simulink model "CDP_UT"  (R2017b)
settings: Solver=FixedStepDiscrete  StartTime=0.0  StopTime=10.0  FixedStep=0.01  RelTol=1e-3  EnableMultiTasking=on
undefined symbols (not defined in the file): ASWTYPE_FALSE, ASWTYPE_TRUE, CaCDP_CellTempNTCVoltTable_mV, CaCDP_CellTempTable_C, CaCDP_CMUPCBTempNTCVoltTable_mV, CaCDP_CMUPCBTempTable_C, CbCDP_DiffBusbarTempStateCheck_flg, CbCDP_DiffCellTempStateCheck_flg, CbCDP_DiffCellVoltStateCheck_flg, CbCDP_IgnorUpdateVld_flg, CbCDP_MaxBusbarTempStateCheck_flg, CbCDP_MaxCellTempStateCheck_flg, CbCDP_MaxCellVoltStateCheck_flg, CbCDP_MinBusbarTempStateCheck_flg, CbCDP_MinCellTempStateCheck_flg, CbCDP_MinCellVoltStateCheck_flg, CcCDP_AFETempConfig_numb, CcCDP_AFETempFltThd_C, CcCDP_AFETempFltThdHys_C, CcCDP_BusbarTempRngFltHiThrd_C, CcCDP_BusbarTempRngFltLowThrd_C, CcCDP_CellDiffFltLevel1_mV, CcCDP_CellDiffFltLevel2_mV, CcCDP_CellDiffFltLevel3_mV, CcCDP_CellTempLowerLimit_C, CcCDP_CellTempRngFltHiThrd_C, CcCDP_CellTempRngFltLowThrd_C, CcCDP_CellTempUpperLimit_C, CcCDP_CellVoltConfig_numb, CcCDP_CellVoltLowerLimit_mV, CcCDP_CellVoltRngHiThrd_mV, CcCDP_CellVoltRngLowThrd_mV, CcCDP_CellVoltUpdateThrd_numb, CcCDP_CellVoltUpperLimit_mV, CcCDP_ChrgMaxCellTempFltLv1Thrd_C, CcCDP_ChrgMaxCellTempFltLv2Thrd_C, CcCDP_ChrgMaxCellTempFltLv3Thrd_C, CcCDP_ChrgMaxCellTempReturnDiff_C, CcCDP_ChrgMinCellTempFltLv1Thrd_C, CcCDP_ChrgMinCellTempFltLv2Thrd_C, CcCDP_ChrgMinCellTempFltLv3Thrd_C, CcCDP_ChrgMinCellTempReturnDiff_C, CcCDP_CMUPCBTempConfig_numb, CcCDP_CMUPCBTempFltThd_C, CcCDP_CMUPCBTempFltThdHys_C, CcCDP_DiffBusbarTempFltLevel1Thrd_C, CcCDP_DiffBusbarTempFltLevel2Thrd_C, CcCDP_DiffBusbarTempReturnDifference_C, CcCDP_DiffCellTempFltLevel1Thrd_C, CcCDP_DiffCellTempFltLevel2Thrd_C, CcCDP_DiffCellTempReturnDifference_C, CcCDP_DiffCellVoltReturnDifference_mV, CcCDP_DiffVoltCheckMaxCellTempCondition_C, CcCDP_DiffVoltCheckMaxCellVoltCondition_mV, CcCDP_DiffVoltCheckMinCellTempCondition_C, CcCDP_DiffVoltCheckMinCellVoltCondition_mV, CcCDP_DiffVoltCheckPackCurrCondition_A, CcCDP_MaxAFETempIniVal_C, CcCDP_MaxBusbarTempFltLevel1Thrd_C, CcCDP_MaxBusbarTempFltLevel2Thrd_C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
libraries: AIWAYS_Powertrain_BMS_lib x148, simulink x8
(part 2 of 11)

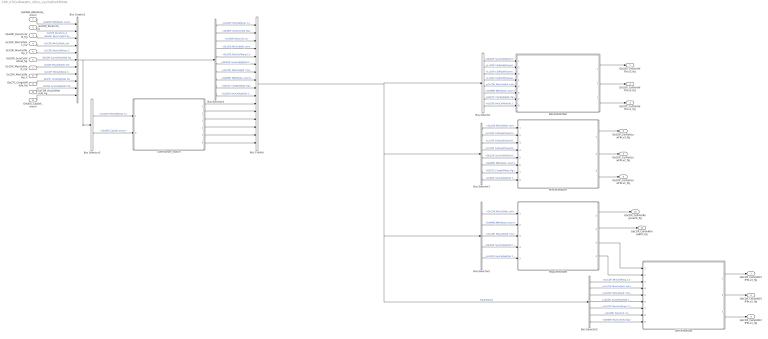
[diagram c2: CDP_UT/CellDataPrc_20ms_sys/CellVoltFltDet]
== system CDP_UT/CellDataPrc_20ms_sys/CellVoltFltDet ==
  GeMSM_BMUState_enum : Inport
  GcHDP_PackCrnt_A : Inport  Port=2
  GbHDP_PackCrntVld_flg : Inport  Port=3
  GcCDP_MinCellVolt_mV : Inport  Port=4
  GcCDP_MaxCellTemp_C : Inport  Port=5
  GbCDP_SumCellVoltVld_flg : Inport  Port=6
  GcCDP_MaxCellVolt_mV : Inport  Port=7
  GcCDP_MinCellTemp_C : Inport  Port=8
  GbCTC_ChrgHVMode_flg : Inport  Port=9
  LbCDP_AnyCellVoltVld_flg : Inport  Port=10
  GeUDS_CapSel_enum : Inport  Port=11
  Bus Creator : BusCreator  Inputs=16
  Bus Creator1 : BusCreator  Inputs=11
  Bus Selector : BusSelector  OutputSignals=GbCDP_SumCellVoltVld_flg,LcCDP_CellHighFltLevel1_mV,LcCDP_CellHighFltLevel2_mV,LcCDP_CellHighFltLevel3_mV,GcCDP_MaxCellVolt_mV,GeMSM_BMUState_enum,GbCTC_ChrgHVMode_flg,LbCDP_AnyCellVoltVld_flg
  Bus Selector1 : BusSelector  OutputSignals=GcCDP_MinCellVolt_mV,LcCDP_CellLowFltLevel1_mV,LcCDP_CellLowFltLevel2_mV,LcCDP_CellLowFltLevel3_mV,GbCDP_SumCellVoltVld_flg,GeMSM_BMUState_enum,GbCTC_ChrgHVMode_flg,LbCDP_AnyCellVoltVld_flg
  Bus Selector2 : BusSelector  OutputSignals=GcCDP_MinCellTemp_C,GcCDP_MaxCellVolt_mV,GcCDP_MinCellVolt_mV,LbCDP_AnyCellVoltVld_flg,GcCDP_MaxCellTemp_C,GcHDP_PackCrnt_A,GbHDP_PackCrntVld_flg
  Bus Selector3 : BusSelector  OutputSignals=GcCDP_MinCellTemp_C,GeUDS_CapSel_enum
  Bus Selector4 : BusSelector  OutputSignals=GcCDP_MinCellTemp_C,GbHDP_PackCrntVld_flg,GcHDP_PackCrnt_A,GcCDP_MinCellVolt_mV,GcCDP_MaxCellTemp_C,GbCDP_SumCellVoltVld_flg,GcCDP_MaxCellVolt_mV,GeMSM_BMUState_enum,GbCTC_ChrgHVMode_flg,LbCDP_AnyCellVoltVld_flg
  Bus Selector5 : BusSelector  OutputSignals=GcCDP_MinCellVolt_mV,GeMSM_BMUState_enum,GcCDP_MaxCellVolt_mV,GbCDP_SumCellVoltVld_flg,LbCDP_AnyCellVoltVld_flg
  CellFltLevel_Switch : Subsystem
  DiffCellVoltDet : Subsystem
  MaxCellVoltDet : Subsystem
  MinCellVoltDet : Subsystem
  RngCellVoltDet : Subsystem
  GbCDP_CellVoltHiFltLv3_flg : Outport
  GbCDP_CellVoltHiFltLv2_flg : Outport  Port=2
  GbCDP_CellVoltHiFltLv1_flg : Outport  Port=3
  GbCDP_CellVoltLowFltLv3_flg : Outport  Port=4
  GbCDP_CellVoltLowFltLv2_flg : Outport  Port=5
  GbCDP_CellVoltLowFltLv1_flg : Outport  Port=6
  GbCDP_CellVoltDiffFltLv3_flg : Outport  Port=7
  GbCDP_CellVoltDiffFltLv2_flg : Outport  Port=8
  GbCDP_CellVoltDiffFltLv1_flg : Outport  Port=9
  GbCDP_CellVoltRngLowFlt_flg : Outport  Port=10
  GbCDP_CellVoltRngHiFlt_flg : Outport  Port=11
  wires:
  Bus Selector4/7 -> Bus Creator/7  "<GcCDP_MaxCellVolt_mV>"
  CellFltLevel_Switch/4(LcCDP_CellLowFltLevel1_mV) -> Bus Creator/14
  CellFltLevel_Switch/2(LcCDP_CellHighFltLevel2_mV) -> Bus Creator/12
  Bus Creator1/1 -> Bus Selector3/1, Bus Selector4/1
  Bus Selector4/3 -> Bus Creator/3  "<GcHDP_PackCrnt_A>"
  Bus Selector4/2 -> Bus Creator/2  "<GbHDP_PackCrntVld_flg>"
  CellFltLevel_Switch/6(LcCDP_CellLowFltLevel3_mV) -> Bus Creator/16
  Bus Selector4/5 -> Bus Creator/5  "<GcCDP_MaxCellTemp_C>"
  CellFltLevel_Switch/1(LcCDP_CellHighFltLevel1_mV) -> Bus Creator/11
  Bus Selector4/8 -> Bus Creator/8  "<GeMSM_BMUState_enum>"
  CellFltLevel_Switch/3(LcCDP_CellHighFltLevel3_mV) -> Bus Creator/13
  Bus Selector4/4 -> Bus Creator/4  "<GcCDP_MinCellVolt_mV>"
  Bus Creator/1 -> Bus Selector2/1, Bus Selector5/1, Bus Selector1/1, Bus Selector/1  "InputSignals"
  Bus Selector3/1 -> CellFltLevel_Switch/1(GcCDP_MinCellTemp_C)  "<GcCDP_MinCellTemp_C>"
  Bus Selector4/1 -> Bus Creator/1  "<GcCDP_MinCellTemp_C>"
  CellFltLevel_Switch/5(LcCDP_CellLowFltLevel2_mV) -> Bus Creator/15
  Bus Selector4/6 -> Bus Creator/6  "<GbCDP_SumCellVoltVld_flg>"
  GeMSM_BMUState_enum/1 -> Bus Creator1/1  "GeMSM_BMUState_enum"
  GcHDP_PackCrnt_A/1 -> Bus Creator1/2  "GcHDP_PackCrnt_A"
  GbHDP_PackCrntVld_flg/1 -> Bus Creator1/3  "GbHDP_PackCrntVld_flg"
  GcCDP_MinCellVolt_mV/1 -> Bus Creator1/4  "GcCDP_MinCellVolt_mV"
  GcCDP_MaxCellTemp_C/1 -> Bus Creator1/5  "GcCDP_MaxCellTemp_C"
  GbCDP_SumCellVoltVld_flg/1 -> Bus Creator1/6  "GbCDP_SumCellVoltVld_flg"
  GcCDP_MaxCellVolt_mV/1 -> Bus Creator1/7  "GcCDP_MaxCellVolt_mV"
  GcCDP_MinCellTemp_C/1 -> Bus Creator1/8  "GcCDP_MinCellTemp_C"
  GbCTC_ChrgHVMode_flg/1 -> Bus Creator1/9  "GbCTC_ChrgHVMode_flg"
  Bus Selector4/9 -> Bus Creator/9  "<GbCTC_ChrgHVMode_flg>"
  MaxCellVoltDet/1(GbCDP_CellVoltHiFltLv3_flg) -> GbCDP_CellVoltHiFltLv3_flg/1
  MaxCellVoltDet/2(GbCDP_CellVoltHiFltLv2_flg) -> GbCDP_CellVoltHiFltLv2_flg/1
  MaxCellVoltDet/3(GbCDP_CellVoltHiFltLv1_flg) -> GbCDP_CellVoltHiFltLv1_flg/1
  MinCellVoltDet/1(GbCDP_CellVoltLowFltLv3_flg) -> GbCDP_CellVoltLowFltLv3_flg/1
  MinCellVoltDet/2(GbCDP_CellVoltLowFltLv2_flg) -> GbCDP_CellVoltLowFltLv2_flg/1
  MinCellVoltDet/3(GbCDP_CellVoltLowFltLv1_flg) -> GbCDP_CellVoltLowFltLv1_flg/1
  DiffCellVoltDet/1(GbCDP_CellVoltDiffFltLv3_flg) -> GbCDP_CellVoltDiffFltLv3_flg/1
  DiffCellVoltDet/2(GbCDP_CellVoltDiffFltLv2_flg) -> GbCDP_CellVoltDiffFltLv2_flg/1
  DiffCellVoltDet/3(GbCDP_CellVoltDiffFltLv1_flg) -> GbCDP_CellVoltDiffFltLv1_flg/1
  Bus Selector5/1 -> RngCellVoltDet/1(GcCDP_MinCellVolt_mV)  "<GcCDP_MinCellVolt_mV>"
  Bus Selector5/2 -> RngCellVoltDet/2(GeMSM_BMUState_enum)  "<GeMSM_BMUState_enum>"
  Bus Selector5/3 -> RngCellVoltDet/3(GcCDP_MaxCellVolt_mV)  "<GcCDP_MaxCellVolt_mV>"
  Bus Selector5/4 -> RngCellVoltDet/4(GbCDP_SumCellVoltVld_flg)  "<GbCDP_SumCellVoltVld_flg>"
  RngCellVoltDet/1(GbCDP_CellVoltRngLowFlt_flg) -> GbCDP_CellVoltRngLowFlt_flg/1
  RngCellVoltDet/2(GbCDP_CellVoltRngHiFlt_flg) -> GbCDP_CellVoltRngHiFlt_flg/1
  LbCDP_AnyCellVoltVld_flg/1 -> Bus Creator1/10  "LbCDP_AnyCellVoltVld_flg"
  Bus Selector4/10 -> Bus Creator/10  "<LbCDP_AnyCellVoltVld_flg>"
  Bus Selector5/5 -> RngCellVoltDet/5(LbCDP_AnyCellVoltVld_flg)  "<LbCDP_AnyCellVoltVld_flg>"
  Bus Selector/1 -> MaxCellVoltDet/1(GbCDP_SumCellVoltVld_flg)  "<GbCDP_SumCellVoltVld_flg>"
  Bus Selector/2 -> MaxCellVoltDet/2(LcCDP_CellHighFltLevel1_mV)  "<LcCDP_CellHighFltLevel1_mV>"
  Bus Selector/3 -> MaxCellVoltDet/3(LcCDP_CellHighFltLevel2_mV)  "<LcCDP_CellHighFltLevel2_mV>"
  Bus Selector/4 -> MaxCellVoltDet/4(LcCDP_CellHighFltLevel3_mV)  "<LcCDP_CellHighFltLevel3_mV>"
  Bus Selector/5 -> MaxCellVoltDet/5(GcCDP_MaxCellVolt_mV)  "<GcCDP_MaxCellVolt_mV>"
  Bus Selector/6 -> MaxCellVoltDet/6(GeMSM_BMUState_enum)  "<GeMSM_BMUState_enum>"
  Bus Selector/7 -> MaxCellVoltDet/7(GbCTC_ChrgHVMode_flg)  "<GbCTC_ChrgHVMode_flg>"
  Bus Selector/8 -> MaxCellVoltDet/8(LbCDP_AnyCellVoltVld_flg)  "<LbCDP_AnyCellVoltVld_flg>"
  Bus Selector1/1 -> MinCellVoltDet/1(GcCDP_MinCellVolt_mV)  "<GcCDP_MinCellVolt_mV>"
  Bus Selector1/2 -> MinCellVoltDet/2(LcCDP_CellLowFltLevel1_mV)  "<LcCDP_CellLowFltLevel1_mV>"
  Bus Selector1/3 -> MinCellVoltDet/3(LcCDP_CellLowFltLevel2_mV)  "<LcCDP_CellLowFltLevel2_mV>"
  Bus Selector1/4 -> MinCellVoltDet/4(LcCDP_CellLowFltLevel3_mV)  "<LcCDP_CellLowFltLevel3_mV>"
  Bus Selector1/5 -> MinCellVoltDet/5(GbCDP_SumCellVoltVld_flg)  "<GbCDP_SumCellVoltVld_flg>"
  Bus Selector1/6 -> MinCellVoltDet/6(GeMSM_BMUState_enum)  "<GeMSM_BMUState_enum>"
  Bus Selector1/7 -> MinCellVoltDet/7(GbCTC_ChrgHVMode_flg)  "<GbCTC_ChrgHVMode_flg>"
  Bus Selector1/8 -> MinCellVoltDet/8(LbCDP_AnyCellVoltVld_flg)  "<LbCDP_AnyCellVoltVld_flg>"
  Bus Selector2/1 -> DiffCellVoltDet/3(GcCDP_MinCellTemp_C)  "<GcCDP_MinCellTemp_C>"
  Bus Selector2/2 -> DiffCellVoltDet/4(GcCDP_MaxCellVolt_mV)  "<GcCDP_MaxCellVolt_mV>"
  Bus Selector2/3 -> DiffCellVoltDet/5(GcCDP_MinCellVolt_mV)  "<GcCDP_MinCellVolt_mV>"
  Bus Selector2/4 -> DiffCellVoltDet/6(LbCDP_AnyCellVoltVld_flg)  "<LbCDP_AnyCellVoltVld_flg>"
  Bus Selector2/5 -> DiffCellVoltDet/7(GcCDP_MaxCellTemp_C)  "<GcCDP_MaxCellTemp_C>"
  Bus Selector2/6 -> DiffCellVoltDet/8(GcHDP_PackCrnt_A)  "<GcHDP_PackCrnt_A>"
  Bus Selector2/7 -> DiffCellVoltDet/9(GbHDP_PackCrntVld_flg)  "<GbHDP_PackCrntVld_flg>"
  RngCellVoltDet/3(LbCDP_CellVoltRngLowFlt_flg) -> DiffCellVoltDet/1(LbCDP_CellVoltRngLowFlt_flg)
  RngCellVoltDet/4(LbCDP_CellVoltRngHiFlt_flg) -> DiffCellVoltDet/2(LbCDP_CellVoltRngHiFlt_flg)
  GeUDS_CapSel_enum/1 -> Bus Creator1/11
  Bus Selector3/2 -> CellFltLevel_Switch/2(GeUDS_CapSel_enum)  "<GeUDS_CapSel_enum>"

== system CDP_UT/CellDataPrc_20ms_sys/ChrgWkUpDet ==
  GeCTC_CtrCtlConnMode_enum : Inport
  Comparison1 : RelationalOperator  Operator===  OutDataTypeStr=boolean
  Comparison2 : RelationalOperator  Operator===  OutDataTypeStr=boolean
  Constant2 : Constant  Value=Enum_CTCCtrCtlConnMode.Enum_CTCCtrCtlConnMode_ACChrg
  Constant3 : Constant  Value=Enum_CTCCtrCtlConnMode.Enum_CTCCtrCtlConnMode_DCChrg
  Data Type Conversion : DataTypeConversion
  Logical1 : Logic  Operator=OR  OutDataTypeStr=boolean
  LbCDP_ChrgWkUp_flg : Outport
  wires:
  GeCTC_CtrCtlConnMode_enum/1 -> Data Type Conversion/1
  Constant2/1 -> Comparison1/2
  Logical1/1 -> LbCDP_ChrgWkUp_flg/1  "LbCDP_ChrgWkUp_flg"
  Constant3/1 -> Comparison2/1
  Comparison2/1 -> Logical1/1
  Comparison1/1 -> Logical1/2
  Data Type Conversion/1 -> Comparison1/1, Comparison2/2

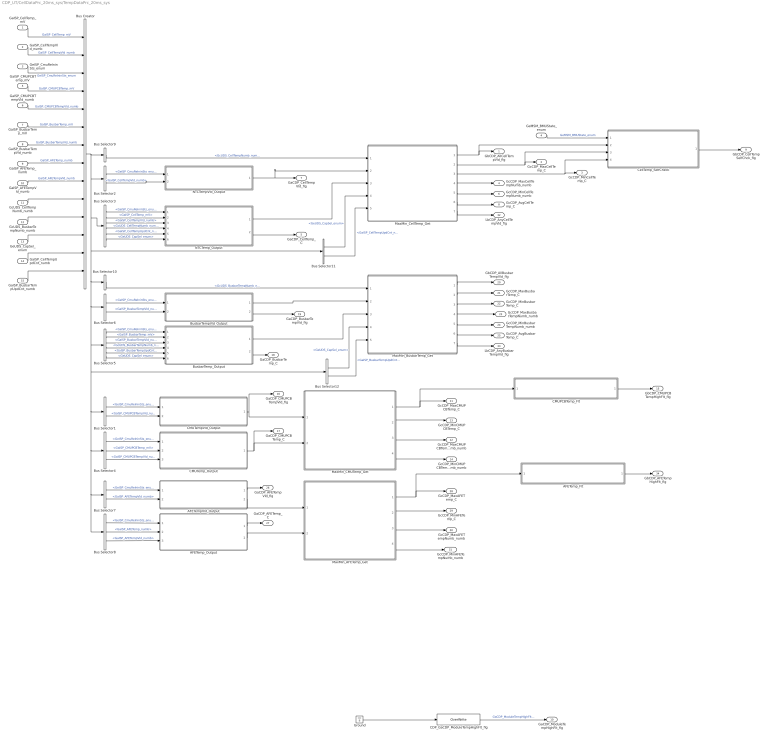
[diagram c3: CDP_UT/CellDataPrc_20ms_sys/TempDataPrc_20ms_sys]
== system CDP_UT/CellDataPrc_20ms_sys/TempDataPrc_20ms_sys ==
  GaISP_CellTemp_mV : Inport
  GaISP_CellTempVld_numb : Inport  Port=2
  GeISP_CmuReIninSts_enum : Inport  Port=3
  GeMSM_BMUState_enum : Inport  Port=4
  GaISP_CMUPCBTemp_mV : Inport  Port=5
  GaISP_CMUPCBTempVld_numb : Inport  Port=6
  GaISP_BusbarTemp_mV : Inport  Port=7
  GaISP_BusbarTempVld_numb : Inport  Port=8
  GaISP_AFETemp_numb : Inport  Port=9
  GaISP_AFETempVld_numb : Inport  Port=10
  GcUDS_CellTempNumb_numb : Inport  Port=11
  GcUDS_BusbarTempNumb_numb : Inport  Port=12
  GeUDS_CapSel_enum : Inport  Port=13
  GaISP_CellTempUpdCnt_numb : Inport  Port=14
  GaISP_BusbarTempUpdCnt_numb : Inport  Port=15
  AFETempVld_Output : Subsystem
  AFETemp_Flt : Subsystem
  AFETemp_Output : Subsystem
  Bus Creator : BusCreator  Inputs=14
  Bus Selector1 : BusSelector  OutputSignals=GeISP_CmuReIninSts_enum,GaISP_CMUPCBTempVld_numb
  Bus Selector10 : BusSelector  OutputSignals=GcUDS_BusbarTempNumb_numb
  Bus Selector11 : BusSelector  OutputSignals=GeUDS_CapSel_enum,GaISP_CellTempUpdCnt_numb
  Bus Selector12 : BusSelector  OutputSignals=GeUDS_CapSel_enum,GaISP_BusbarTempUpdCnt_numb
  Bus Selector2 : BusSelector  OutputSignals=GeISP_CmuReIninSts_enum,GaISP_CellTempVld_numb
  Bus Selector3 : BusSelector  OutputSignals=GeISP_CmuReIninSts_enum,GaISP_CellTemp_mV,GaISP_CellTempVld_numb,GcUDS_CellTempNumb_numb,GaISP_CellTempUpdCnt_numb,GeUDS_CapSel_enum
  Bus Selector4 : BusSelector  OutputSignals=GeISP_CmuReIninSts_enum,GaISP_CMUPCBTemp_mV,GaISP_CMUPCBTempVld_numb
  Bus Selector5 : BusSelector  OutputSignals=GeISP_CmuReIninSts_enum,GaISP_BusbarTemp_mV,GaISP_BusbarTempVld_numb,GcUDS_BusbarTempNumb_numb,GaISP_BusbarTempUpdCnt_numb,GeUDS_CapSel_enum
  Bus Selector6 : BusSelector  OutputSignals=GeISP_CmuReIninSts_enum,GaISP_BusbarTempVld_numb
  Bus Selector7 : BusSelector  OutputSignals=GeISP_CmuReIninSts_enum,GaISP_AFETempVld_numb
  Bus Selector8 : BusSelector  OutputSignals=GeISP_CmuReIninSts_enum,GaISP_AFETemp_numb,GaISP_AFETempVld_numb
  Bus Selector9 : BusSelector  OutputSignals=GcUDS_CellTempNumb_numb
  BusbarTempVld_Output : Subsystem
  BusbarTemp_Output : Subsystem
  CDP_GaCDP_ModuleTempHighFlt_flg : AIWAYS_Powertrain_BMS_lib/Signals/OverWrite  OverWrite_Value=CaCDP_ModuleTempHighFltOvr_flg  OverWrite_flag=CbCDP_ModuleTempHighFltOvrSwt_flg
  CMUPCBTemp_Flt : Subsystem
  CMUTempVld_Output : Subsystem
  CMUTemp_Output : Subsystem
  CellTemp_SelfCheck : Subsystem
  Ground : Ground
  MaxMin_AFETemp_Get : Subsystem
  MaxMin_BusbarTemp_Get : Subsystem
  MaxMin_CMUTemp_Get : Subsystem
  MaxMin_CellTemp_Get : Subsystem
  NTCTempVld_Output : Subsystem
  NTCTemp_Output : Subsystem
  GbCDP_AllCellTempVld_flg : Outport
  GcCDP_MaxCellTemp_C : Outport  Port=2
  GcCDP_MinCellTemp_C : Outport  Port=3
  GcCDP_MaxCellTempNumb_numb : Outport  Port=4
  GaCDP_CellTemp_C : Outport  Port=5
  GcCDP_MinCellTempNumb_numb : Outport  Port=6
  GaCDP_CellTempVld_flg : Outport  Port=7
  GcCDP_AvgCellTemp_C : Outport  Port=8
  GbCDP_CellTempSelfChck_flg : Outport  Port=9
  GaCDP_ModuleTempHighFlt_flg : Outport  Port=10
  GcCDP_MaxCMUPCBTemp_C : Outport  Port=11
  GcCDP_MaxCMUPCBTempNumb_numb : Outport  Port=12
  GcCDP_MinCMUPCBTemp_C : Outport  Port=13
  GcCDP_MinCMUPCBTempNumb_numb : Outport  Port=14
  GbCDP_CMUPCBTempHighFlt_flg : Outport  Port=15
  GaCDP_CMUPCBTempVld_flg : Outport  Port=16
  GaCDP_CMUPCBTemp_C : Outport  Port=17
  GaCDP_BusbarTemp_C : Outport  Port=18
  GaCDP_BusbarTempVld_flg : Outport  Port=19
  GbCDP_AllBusbarTempVld_flg : Outport  Port=20
  GcCDP_MaxBusbarTemp_C : Outport  Port=21
  GcCDP_MinBusbarTemp_C : Outport  Port=22
  GcCDP_MaxBusbarTempNumb_numb : Outport  Port=23
  GcCDP_MinBusbarTempNumb_numb : Outport  Port=24
  GcCDP_AvgBusbarTemp_C : Outport  Port=25
  GaCDP_AFETempVld_flg : Outport  Port=26
  GaCDP_AFETemp_C : Outport  Port=27
  GcCDP_MaxAFETemp_C : Outport  Port=28
  GcCDP_MinAFETemp_C : Outport  Port=29
  GcCDP_MaxAFETempNumb_numb : Outport  Port=30
  GcCDP_MinAFETempNumb_numb : Outport  Port=31
  LbCDP_AnyCellTempVld_flg : Outport  Port=32
  LbCDP_AnyBusbarTempVld_flg : Outport  Port=33
  GbCDP_AFETempHighFlt_flg : Outport  Port=34
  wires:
  GaISP_CellTemp_mV/1 -> Bus Creator/1  "GaISP_CellTemp_mV"
  GeISP_CmuReIninSts_enum/1 -> Bus Creator/3  "GeISP_CmuReIninSts_enum"
  MaxMin_CellTemp_Get/5(GcCDP_MinCellTempNumb_numb) -> GcCDP_MinCellTempNumb_numb/1
  MaxMin_CellTemp_Get/6(GcCDP_AvgCellTemp_C) -> GcCDP_AvgCellTemp_C/1
  GaISP_CellTempVld_numb/1 -> Bus Creator/2  "GaISP_CellTempVld_numb"
  MaxMin_CellTemp_Get/3(GcCDP_MinCellTemp_C) -> CellTemp_SelfCheck/4(GcCDP_MinCellTemp_C), GcCDP_MinCellTemp_C/1
  MaxMin_CellTemp_Get/2(GcCDP_MaxCellTemp_C) -> CellTemp_SelfCheck/3(GcCDP_MaxCellTemp_C), GcCDP_MaxCellTemp_C/1
  MaxMin_CellTemp_Get/1(GbCDP_AllCellTempVld_flg) -> CellTemp_SelfCheck/2(GbCDP_AllCellTempVld_flg), GbCDP_AllCellTempVld_flg/1
  MaxMin_CellTemp_Get/4(GcCDP_MaxCellTempNumb_numb) -> GcCDP_MaxCellTempNumb_numb/1
  NTCTempVld_Output/1(GaCDP_CellTempVld_flg) -> MaxMin_CellTemp_Get/2(GaCDP_CellTempVld_flg), GaCDP_CellTempVld_flg/1
  Bus Selector2/1 -> NTCTempVld_Output/1(GeISP_CmuReIninSts_enum)  "<GeISP_CmuReIninSts_enum>"
  Bus Selector2/2 -> NTCTempVld_Output/2(GaISP_CellTempVld_numb)  "<GaISP_CellTempVld_numb>"
  Bus Selector3/2 -> NTCTemp_Output/2(GaISP_CellTemp_mV)  "<GaISP_CellTemp_mV>"
  Bus Selector3/1 -> NTCTemp_Output/1(GeISP_CmuReIninSts_enum)  "<GeISP_CmuReIninSts_enum>"
  Bus Selector3/3 -> NTCTemp_Output/3(GaISP_CellTempVld_numb)  "<GaISP_CellTempVld_numb>"
  CellTemp_SelfCheck/1(GbCDP_CellTempSelfChck_flg) -> GbCDP_CellTempSelfChck_flg/1
  GeMSM_BMUState_enum/1 -> CellTemp_SelfCheck/1(GeMSM_BMUState_enum)  "GeMSM_BMUState_enum"
  GaISP_CMUPCBTemp_mV/1 -> Bus Creator/4  "GaISP_CMUPCBTemp_mV"
  GaISP_CMUPCBTempVld_numb/1 -> Bus Creator/5  "GaISP_CMUPCBTempVld_numb"
  CDP_GaCDP_ModuleTempHighFlt_flg/1 -> GaCDP_ModuleTempHighFlt_flg/1  "GaCDP_ModuleTempHighFlt_flg"
  Ground/1 -> CDP_GaCDP_ModuleTempHighFlt_flg/1
  CMUTemp_Output/1(GaCDP_CMUPCBTemp_C) -> MaxMin_CMUTemp_Get/2(GaCDP_CMUPCBTemp_C), GaCDP_CMUPCBTemp_C/1
  Bus Selector1/1 -> CMUTempVld_Output/1(GeISP_CmuReIninSts_enum)  "<GeISP_CmuReIninSts_enum>"
  Bus Selector4/1 -> CMUTemp_Output/1(GeISP_CmuReIninSts_enum)  "<GeISP_CmuReIninSts_enum>"
  Bus Selector4/3 -> CMUTemp_Output/3(GaISP_CMUPCBTempVld_numb)  "<GaISP_CMUPCBTempVld_numb>"
  Bus Selector4/2 -> CMUTemp_Output/2(GaISP_CMUPCBTemp_mV)  "<GaISP_CMUPCBTemp_mV>"
  CMUTempVld_Output/1(GaCDP_CMUPCBTempVld_flg) -> MaxMin_CMUTemp_Get/1(GaCDP_CMUPCBTempVld_flg), GaCDP_CMUPCBTempVld_flg/1
  Bus Selector1/2 -> CMUTempVld_Output/2(GaISP_CMUPCBTempVld_numb)  "<GaISP_CMUPCBTempVld_numb>"
  MaxMin_CMUTemp_Get/1(GcCDP_MaxCMUPCBTemp_C) -> CMUPCBTemp_Flt/1(GcCDP_MaxCMUPCBTemp_C), GcCDP_MaxCMUPCBTemp_C/1
  CMUPCBTemp_Flt/1(GbCDP_CMUPCBTempHighFlt_flg) -> GbCDP_CMUPCBTempHighFlt_flg/1
  MaxMin_CMUTemp_Get/2(GcCDP_MinCMUPCBTemp_C) -> GcCDP_MinCMUPCBTemp_C/1
  MaxMin_CMUTemp_Get/3(GcCDP_MaxCMUPCBTempNumb_numb) -> GcCDP_MaxCMUPCBTempNumb_numb/1
  MaxMin_CMUTemp_Get/4(GcCDP_MinCMUPCBTempNumb_numb) -> GcCDP_MinCMUPCBTempNumb_numb/1
  GaISP_BusbarTemp_mV/1 -> Bus Creator/6  "GaISP_BusbarTemp_mV"
  GaISP_BusbarTempVld_numb/1 -> Bus Creator/7  "GaISP_BusbarTempVld_numb"
  Bus Selector6/1 -> BusbarTempVld_Output/1(GeISP_CmuReIninSts_enum)  "<GeISP_CmuReIninSts_enum>"
  Bus Selector6/2 -> BusbarTempVld_Output/2(GaISP_BusbarTempVld_numb)  "<GaISP_BusbarTempVld_numb>"
  Bus Selector5/1 -> BusbarTemp_Output/1(GeISP_CmuReIninSts_enum)  "<GeISP_CmuReIninSts_enum>"
  Bus Selector5/2 -> BusbarTemp_Output/2(GaISP_BusbarTemp_mV)  "<GaISP_BusbarTemp_mV>"
  Bus Selector5/3 -> BusbarTemp_Output/3(GaISP_BusbarTempVld_numb)  "<GaISP_BusbarTempVld_numb>"
  BusbarTemp_Output/1(LaCDP_BusbarTemp_C) -> MaxMin_BusbarTemp_Get/3(LaCDP_BusbarTemp_C)
  BusbarTempVld_Output/2(GaCDP_BusbarTempVld_flg) -> GaCDP_BusbarTempVld_flg/1
  BusbarTemp_Output/2(GaCDP_BusbarTemp_C) -> GaCDP_BusbarTemp_C/1
  BusbarTempVld_Output/1(LaCDP_BusbarTempVld_flg) -> MaxMin_BusbarTemp_Get/2(LaCDP_BusbarTempVld_flg)
  MaxMin_BusbarTemp_Get/1(GbCDP_AllBusbarTempVld_flg) -> GbCDP_AllBusbarTempVld_flg/1
  MaxMin_BusbarTemp_Get/2(GcCDP_MaxBusbarTemp_C) -> GcCDP_MaxBusbarTemp_C/1
  MaxMin_BusbarTemp_Get/3(GcCDP_MinBusbarTemp_C) -> GcCDP_MinBusbarTemp_C/1
  MaxMin_BusbarTemp_Get/4(GcCDP_MaxBusbarTempNumb_numb) -> GcCDP_MaxBusbarTempNumb_numb/1
  MaxMin_BusbarTemp_Get/5(GcCDP_MinBusbarTempNumb_numb) -> GcCDP_MinBusbarTempNumb_numb/1
  MaxMin_BusbarTemp_Get/6(GcCDP_AvgBusbarTemp_C) -> GcCDP_AvgBusbarTemp_C/1
  GaISP_AFETemp_numb/1 -> Bus Creator/8  "GaISP_AFETemp_numb"
  GaISP_AFETempVld_numb/1 -> Bus Creator/9  "GaISP_AFETempVld_numb"
  Bus Selector7/1 -> AFETempVld_Output/1(GeISP_CmuReIninSts_enum)  "<GeISP_CmuReIninSts_enum>"
  Bus Selector7/2 -> AFETempVld_Output/2(GaISP_AFETempVld_numb)  "<GaISP_AFETempVld_numb>"
  Bus Selector8/1 -> AFETemp_Output/1(GeISP_CmuReIninSts_enum)  "<GeISP_CmuReIninSts_enum>"
  Bus Selector8/2 -> AFETemp_Output/2(GaISP_AFETemp_numb)  "<GaISP_AFETemp_numb>"
  Bus Selector8/3 -> AFETemp_Output/3(GaISP_AFETempVld_numb)  "<GaISP_AFETempVld_numb>"
  AFETemp_Output/2(LaCDP_AFETemp_C) -> MaxMin_AFETemp_Get/2(LaCDP_AFETemp_C)
  AFETempVld_Output/2(LaCDP_AFETempVld_flg) -> MaxMin_AFETemp_Get/1(LaCDP_AFETempVld_flg)
  AFETempVld_Output/1(GaCDP_AFETempVld_flg) -> GaCDP_AFETempVld_flg/1
  AFETemp_Output/1(GaCDP_AFETemp_C) -> GaCDP_AFETemp_C/1
  MaxMin_AFETemp_Get/1(GcCDP_MaxAFETemp_C) -> AFETemp_Flt/1(GcCDP_MaxAFETemp_C), GcCDP_MaxAFETemp_C/1
  MaxMin_AFETemp_Get/2(GcCDP_MinAFETemp_C) -> GcCDP_MinAFETemp_C/1
  MaxMin_AFETemp_Get/3(GcCDP_MaxAFETempNumb_numb) -> GcCDP_MaxAFETempNumb_numb/1
  MaxMin_AFETemp_Get/4(GcCDP_MinAFETempNumb_numb) -> GcCDP_MinAFETempNumb_numb/1
  MaxMin_CellTemp_Get/7(LbCDP_AnyCellTempVld_flg) -> LbCDP_AnyCellTempVld_flg/1
  MaxMin_BusbarTemp_Get/7(LbCDP_AnyBusbarTempVld_flg) -> LbCDP_AnyBusbarTempVld_flg/1
  GcUDS_CellTempNumb_numb/1 -> Bus Creator/10
  GcUDS_BusbarTempNumb_numb/1 -> Bus Creator/11
  Bus Creator/1 -> Bus Selector11/1, Bus Selector12/1, Bus Selector8/1, Bus Selector7/1, Bus Selector4/1, Bus Selector1/1, Bus Selector5/1, Bus Selector6/1, Bus Selector10/1, Bus Selector3/1, Bus Selector2/1, Bus Selector9/1
  Bus Selector10/1 -> MaxMin_BusbarTemp_Get/1(GcUDS_BusbarTempNumb_numb)  "<GcUDS_BusbarTempNumb_numb>"
  Bus Selector9/1 -> MaxMin_CellTemp_Get/1(GcUDS_CellTempNumb_numb)  "<GcUDS_CellTempNumb_numb>"
  Bus Selector5/4 -> BusbarTemp_Output/4(GcUDS_BusbarTempNumb_numb)  "<GcUDS_BusbarTempNumb_numb>"
  Bus Selector3/4 -> NTCTemp_Output/4(GcUDS_CellTempNumb_numb)  "<GcUDS_CellTempNumb_numb>"
  AFETemp_Flt/1(GbCDP_AFETempHighFlt_flg) -> GbCDP_AFETempHighFlt_flg/1
  GeUDS_CapSel_enum/1 -> Bus Creator/12
  GaISP_CellTempUpdCnt_numb/1 -> Bus Creator/13
  Bus Selector11/1 -> MaxMin_CellTemp_Get/4(GeUDS_CapSel_enum)  "<GeUDS_CapSel_enum>"
  Bus Selector11/2 -> MaxMin_CellTemp_Get/5(GaISP_CellTempUpdCnt_numb)  "<GaISP_CellTempUpdCnt_numb>"
  NTCTemp_Output/1(LaCDP_CellTemp_C) -> MaxMin_CellTemp_Get/3(LaCDP_CellTemp_C)
  NTCTemp_Output/2(GaCDP_CellTemp_C) -> GaCDP_CellTemp_C/1
  Bus Selector3/5 -> NTCTemp_Output/5(GaISP_CellTempUpdCnt_numb)  "<GaISP_CellTempUpdCnt_numb>"
  Bus Selector3/6 -> NTCTemp_Output/6(GeUDS_CapSel_enum)  "<GeUDS_CapSel_enum>"
  GaISP_BusbarTempUpdCnt_numb/1 -> Bus Creator/14
  Bus Selector5/5 -> BusbarTemp_Output/5(GaISP_BusbarTempUpdCnt_numb)  "<GaISP_BusbarTempUpdCnt_numb>"
  Bus Selector5/6 -> BusbarTemp_Output/6(GeUDS_CapSel_enum)  "<GeUDS_CapSel_enum>"
  Bus Selector12/1 -> MaxMin_BusbarTemp_Get/4(GeUDS_CapSel_enum)  "<GeUDS_CapSel_enum>"
  Bus Selector12/2 -> MaxMin_BusbarTemp_Get/5(GaISP_BusbarTempUpdCnt_numb)  "<GaISP_BusbarTempUpdCnt_numb>"

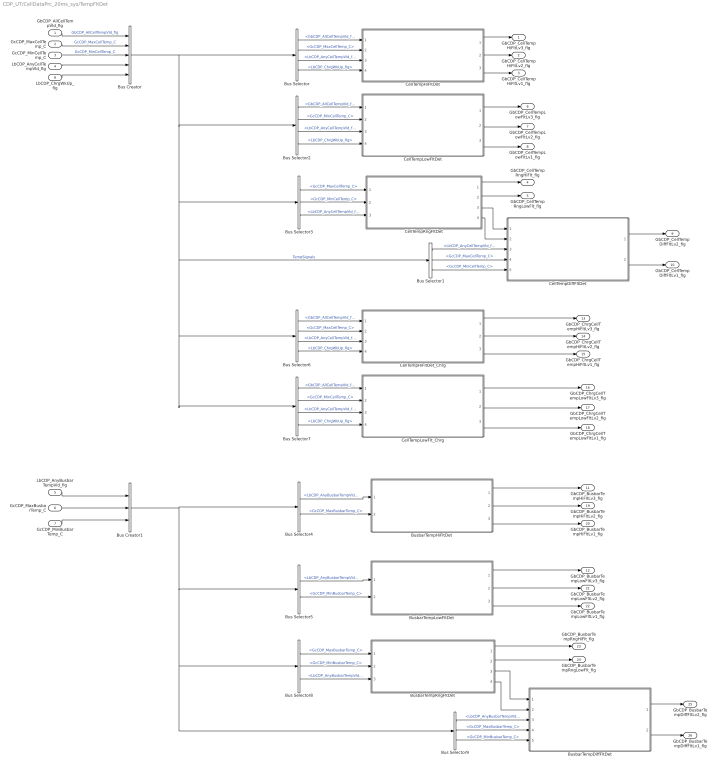
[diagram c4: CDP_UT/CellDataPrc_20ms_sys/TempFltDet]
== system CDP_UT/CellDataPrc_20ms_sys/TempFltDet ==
  GbCDP_AllCellTempVld_flg : Inport
  GcCDP_MaxCellTemp_C : Inport  Port=2
  GcCDP_MinCellTemp_C : Inport  Port=3
  LbCDP_AnyCellTempVld_flg : Inport  Port=4
  LbCDP_AnyBusbarTempVld_flg : Inport  Port=5
  GcCDP_MaxBusbarTemp_C : Inport  Port=6
  GcCDP_MinBusbarTemp_C : Inport  Port=7
  LbCDP_ChrgWkUp_flg : Inport  Port=8
  Bus Creator : BusCreator  Inputs=5
  Bus Creator1 : BusCreator  Inputs=3
  Bus Selector : BusSelector  OutputSignals=GbCDP_AllCellTempVld_flg,GcCDP_MaxCellTemp_C,LbCDP_AnyCellTempVld_flg,LbCDP_ChrgWkUp_flg
  Bus Selector1 : BusSelector  OutputSignals=LbCDP_AnyCellTempVld_flg,GcCDP_MaxCellTemp_C,GcCDP_MinCellTemp_C
  Bus Selector2 : BusSelector  OutputSignals=GbCDP_AllCellTempVld_flg,GcCDP_MinCellTemp_C,LbCDP_AnyCellTempVld_flg,LbCDP_ChrgWkUp_flg
  Bus Selector3 : BusSelector  OutputSignals=GcCDP_MaxCellTemp_C,GcCDP_MinCellTemp_C,LbCDP_AnyCellTempVld_flg
  Bus Selector4 : BusSelector  OutputSignals=LbCDP_AnyBusbarTempVld_flg,GcCDP_MaxBusbarTemp_C
  Bus Selector5 : BusSelector  OutputSignals=LbCDP_AnyBusbarTempVld_flg,GcCDP_MinBusbarTemp_C
  Bus Selector6 : BusSelector  OutputSignals=GbCDP_AllCellTempVld_flg,GcCDP_MaxCellTemp_C,LbCDP_AnyCellTempVld_flg,LbCDP_ChrgWkUp_flg
  Bus Selector7 : BusSelector  OutputSignals=GbCDP_AllCellTempVld_flg,GcCDP_MinCellTemp_C,LbCDP_AnyCellTempVld_flg,LbCDP_ChrgWkUp_flg
  Bus Selector8 : BusSelector  OutputSignals=GcCDP_MaxBusbarTemp_C,GcCDP_MinBusbarTemp_C,LbCDP_AnyBusbarTempVld_flg
  Bus Selector9 : BusSelector  OutputSignals=LbCDP_AnyBusbarTempVld_flg,GcCDP_MaxBusbarTemp_C,GcCDP_MinBusbarTemp_C
  BusbarTempDiffFltDet : Subsystem
  BusbarTempHiFltDet : Subsystem
  BusbarTempLowFltDet : Subsystem
  BusbarTempRngFltDet : Subsystem
  CellTempDiffFltDet : Subsystem
  CellTempHiFltDet : Subsystem
  CellTempHiFltDet_Chrg : Subsystem
  CellTempLowFltDet : Subsystem
  CellTempLowFlt_Chrg : Subsystem
  CellTempRngFltDet : Subsystem
  GbCDP_CellTempHiFltLv3_flg : Outport
  GbCDP_CellTempHiFltLv2_flg : Outport  Port=2
  GbCDP_CellTempHiFltLv1_flg : Outport  Port=3
  GbCDP_CellTempRngHiFlt_flg : Outport  Port=4
  GbCDP_CellTempRngLowFlt_flg : Outport  Port=5
  GbCDP_CellTempLowFltLv3_flg : Outport  Port=6
  GbCDP_CellTempLowFltLv2_flg : Outport  Port=7
  GbCDP_CellTempLowFltLv1_flg : Outport  Port=8
  GbCDP_CellTempDiffFltLv2_flg : Outport  Port=9
  GbCDP_CellTempDiffFltLv1_flg : Outport  Port=10
  GbCDP_BusbarTempHiFltLv3_flg : Outport  Port=11
  GbCDP_BusbarTempLowFltLv3_flg : Outport  Port=12
  GbCDP_ChrgCellTempHiFltLv3_flg : Outport  Port=13
  GbCDP_ChrgCellTempHiFltLv2_flg : Outport  Port=14
  GbCDP_ChrgCellTempHiFltLv1_flg : Outport  Port=15
  GbCDP_ChrgCellTempLowFltLv3_flg : Outport  Port=16
  GbCDP_ChrgCellTempLowFltLv2_flg : Outport  Port=17
  GbCDP_ChrgCellTempLowFltLv1_flg : Outport  Port=18
  GbCDP_BusbarTempHiFltLv2_flg : Outport  Port=19
  GbCDP_BusbarTempHiFltLv1_flg : Outport  Port=20
  GbCDP_BusbarTempLowFltLv2_flg : Outport  Port=21
  GbCDP_BusbarTempLowFltLv1_flg : Outport  Port=22
  GbCDP_BusbarTempRngHiFlt_flg : Outport  Port=23
  GbCDP_BusbarTempRngLowFlt_flg : Outport  Port=24
  GbCDP_BusbarTempDiffFltLv2_flg : Outport  Port=25
  GbCDP_BusbarTempDiffFltLv1_flg : Outport  Port=26
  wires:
  Bus Selector/2 -> CellTempHiFltDet/2(GcCDP_MaxCellTemp_C)  "<GcCDP_MaxCellTemp_C>"
  GcCDP_MaxCellTemp_C/1 -> Bus Creator/2  "GcCDP_MaxCellTemp_C"
  Bus Selector/1 -> CellTempHiFltDet/1(GbCDP_AllCellTempVld_flg)  "<GbCDP_AllCellTempVld_flg>"
  Bus Selector2/1 -> CellTempLowFltDet/1(GbCDP_AllCellTempVld_flg)  "<GbCDP_AllCellTempVld_flg>"
  GbCDP_AllCellTempVld_flg/1 -> Bus Creator/1  "GbCDP_AllCellTempVld_flg"
  GcCDP_MinCellTemp_C/1 -> Bus Creator/3  "GcCDP_MinCellTemp_C"
  Bus Selector2/2 -> CellTempLowFltDet/2(GcCDP_MinCellTemp_C)  "<GcCDP_MinCellTemp_C>"
  CellTempHiFltDet/1(GbCDP_CellTempHiFltLv3_flg) -> GbCDP_CellTempHiFltLv3_flg/1
  CellTempHiFltDet/2(GbCDP_CellTempHiFltLv2_flg) -> GbCDP_CellTempHiFltLv2_flg/1
  CellTempHiFltDet/3(GbCDP_CellTempHiFltLv1_flg) -> GbCDP_CellTempHiFltLv1_flg/1
  Bus Creator/1 -> Bus Selector2/1, Bus Selector7/1, Bus Selector6/1, Bus Selector1/1, Bus Selector3/1, Bus Selector/1  "TempSignals"
  Bus Selector3/1 -> CellTempRngFltDet/1(GcCDP_MaxCellTemp_C)  "<GcCDP_MaxCellTemp_C>"
  Bus Selector3/2 -> CellTempRngFltDet/2(GcCDP_MinCellTemp_C)  "<GcCDP_MinCellTemp_C>"
  CellTempRngFltDet/1(GbCDP_CellTempRngHiFlt_flg) -> GbCDP_CellTempRngHiFlt_flg/1
  CellTempRngFltDet/2(GbCDP_CellTempRngLowFlt_flg) -> GbCDP_CellTempRngLowFlt_flg/1
  Bus Selector2/3 -> CellTempLowFltDet/3(LbCDP_AnyCellTempVld_flg)  "<LbCDP_AnyCellTempVld_flg>"
  CellTempLowFltDet/1(GbCDP_CellTempLowFltLv3_flg) -> GbCDP_CellTempLowFltLv3_flg/1
  CellTempLowFltDet/2(GbCDP_CellTempLowFltLv2_flg) -> GbCDP_CellTempLowFltLv2_flg/1
  CellTempLowFltDet/3(GbCDP_CellTempLowFltLv1_flg) -> GbCDP_CellTempLowFltLv1_flg/1
  CellTempDiffFltDet/1(GbCDP_CellTempDiffFltLv2_flg) -> GbCDP_CellTempDiffFltLv2_flg/1
  CellTempDiffFltDet/2(GbCDP_CellTempDiffFltLv1_flg) -> GbCDP_CellTempDiffFltLv1_flg/1
  LbCDP_AnyCellTempVld_flg/1 -> Bus Creator/4
  Bus Selector/3 -> CellTempHiFltDet/3(LbCDP_AnyCellTempVld_flg)  "<LbCDP_AnyCellTempVld_flg>"
  Bus Selector3/3 -> CellTempRngFltDet/3(LbCDP_AnyCellTempVld_flg)  "<LbCDP_AnyCellTempVld_flg>"
  CellTempRngFltDet/3(LbCDP_CellTempRngHiFlt_flg) -> CellTempDiffFltDet/1(LbCDP_CellTempRngHiFlt_flg)
  CellTempRngFltDet/4(LbCDP_CellTempRngLowFlt_flg) -> CellTempDiffFltDet/2(LbCDP_CellTempRngLowFlt_flg)
  Bus Selector1/1 -> CellTempDiffFltDet/3(LbCDP_AnyCellTempVld_flg)  "<LbCDP_AnyCellTempVld_flg>"
  Bus Selector1/2 -> CellTempDiffFltDet/4(GcCDP_MaxCellTemp_C)  "<GcCDP_MaxCellTemp_C>"
  Bus Selector1/3 -> CellTempDiffFltDet/5(GcCDP_MinCellTemp_C)  "<GcCDP_MinCellTemp_C>"
  LbCDP_AnyBusbarTempVld_flg/1 -> Bus Creator1/1
  GcCDP_MaxBusbarTemp_C/1 -> Bus Creator1/2
  GcCDP_MinBusbarTemp_C/1 -> Bus Creator1/3
  Bus Creator1/1 -> Bus Selector4/1, Bus Selector9/1, Bus Selector8/1, Bus Selector5/1
  Bus Selector4/1 -> BusbarTempHiFltDet/1(LbCDP_AnyBusbarTempVld_flg)  "<LbCDP_AnyBusbarTempVld_flg>"
  Bus Selector4/2 -> BusbarTempHiFltDet/2(GcCDP_MaxBusbarTemp_C)  "<GcCDP_MaxBusbarTemp_C>"
  Bus Selector5/1 -> BusbarTempLowFltDet/1(LbCDP_AnyBusbarTempVld_flg)  "<LbCDP_AnyBusbarTempVld_flg>"
  Bus Selector5/2 -> BusbarTempLowFltDet/2(GcCDP_MinBusbarTemp_C)  "<GcCDP_MinBusbarTemp_C>"
  BusbarTempHiFltDet/1(GbCDP_BusbarTempHiFltLv3_flg) -> GbCDP_BusbarTempHiFltLv3_flg/1
  BusbarTempLowFltDet/1(GbCDP_BusbarTempLowFltLv3_flg) -> GbCDP_BusbarTempLowFltLv3_flg/1
  LbCDP_ChrgWkUp_flg/1 -> Bus Creator/5
  Bus Selector/4 -> CellTempHiFltDet/4(LbCDP_ChrgWkUp_flg)  "<LbCDP_ChrgWkUp_flg>"
  Bus Selector2/4 -> CellTempLowFltDet/4(LbCDP_ChrgWkUp_flg)  "<LbCDP_ChrgWkUp_flg>"
  Bus Selector7/4 -> CellTempLowFlt_Chrg/4(LbCDP_ChrgWkUp_flg)  "<LbCDP_ChrgWkUp_flg>"
  Bus Selector6/4 -> CellTempHiFltDet_Chrg/4(LbCDP_ChrgWkUp_flg)  "<LbCDP_ChrgWkUp_flg>"
  Bus Selector6/3 -> CellTempHiFltDet_Chrg/3(LbCDP_AnyCellTempVld_flg)  "<LbCDP_AnyCellTempVld_flg>"
  Bus Selector7/3 -> CellTempLowFlt_Chrg/3(LbCDP_AnyCellTempVld_flg)  "<LbCDP_AnyCellTempVld_flg>"
  Bus Selector7/2 -> CellTempLowFlt_Chrg/2(GcCDP_MinCellTemp_C)  "<GcCDP_MinCellTemp_C>"
  Bus Selector7/1 -> CellTempLowFlt_Chrg/1(GbCDP_AllCellTempVld_flg)  "<GbCDP_AllCellTempVld_flg>"
  Bus Selector6/1 -> CellTempHiFltDet_Chrg/1(GbCDP_AllCellTempVld_flg)  "<GbCDP_AllCellTempVld_flg>"
  Bus Selector6/2 -> CellTempHiFltDet_Chrg/2(GcCDP_MaxCellTemp_C)  "<GcCDP_MaxCellTemp_C>"
  CellTempHiFltDet_Chrg/1(GbCDP_ChrgCellTempHiFltLv3_flg) -> GbCDP_ChrgCellTempHiFltLv3_flg/1
  CellTempHiFltDet_Chrg/2(GbCDP_ChrgCellTempHiFltLv2_flg) -> GbCDP_ChrgCellTempHiFltLv2_flg/1
  CellTempHiFltDet_Chrg/3(GbCDP_ChrgCellTempHiFltLv1_flg) -> GbCDP_ChrgCellTempHiFltLv1_flg/1
  CellTempLowFlt_Chrg/1(GbCDP_ChrgCellTempLowFltLv3_flg) -> GbCDP_ChrgCellTempLowFltLv3_flg/1
  CellTempLowFlt_Chrg/2(GbCDP_ChrgCellTempLowFltLv2_flg) -> GbCDP_ChrgCellTempLowFltLv2_flg/1
  CellTempLowFlt_Chrg/3(GbCDP_ChrgCellTempLowFltLv1_flg) -> GbCDP_ChrgCellTempLowFltLv1_flg/1
  BusbarTempHiFltDet/2(GbCDP_BusbarTempHiFltLv2_flg) -> GbCDP_BusbarTempHiFltLv2_flg/1
  BusbarTempHiFltDet/3(GbCDP_BusbarTempHiFltLv1_flg) -> GbCDP_BusbarTempHiFltLv1_flg/1
  BusbarTempLowFltDet/2(GbCDP_BusbarTempLowFltLv2_flg) -> GbCDP_BusbarTempLowFltLv2_flg/1
  BusbarTempLowFltDet/3(GbCDP_BusbarTempLowFltLv1_flg) -> GbCDP_BusbarTempLowFltLv1_flg/1
  Bus Selector8/1 -> BusbarTempRngFltDet/1(GcCDP_MaxBusbarTemp_C)  "<GcCDP_MaxBusbarTemp_C>"
  Bus Selector8/2 -> BusbarTempRngFltDet/2(GcCDP_MinBusbarTemp_C)  "<GcCDP_MinBusbarTemp_C>"
  Bus Selector8/3 -> BusbarTempRngFltDet/3(LbCDP_AnyBusbarTempVld_flg)  "<LbCDP_AnyBusbarTempVld_flg>"
  BusbarTempRngFltDet/1(GbCDP_BusbarTempRngHiFlt_flg) -> GbCDP_BusbarTempRngHiFlt_flg/1
  BusbarTempRngFltDet/2(GbCDP_BusbarTempRngLowFlt_flg) -> GbCDP_BusbarTempRngLowFlt_flg/1
  BusbarTempRngFltDet/3(LbCDP_BusbarTempRngHiFlt_flg) -> BusbarTempDiffFltDet/1(LbCDP_BusbarTempRngHiFlt_flg)
  BusbarTempRngFltDet/4(LbCDP_BusbarTempRngLowFlt_flg) -> BusbarTempDiffFltDet/2(LbCDP_BusbarTempRngLowFlt_flg)
  Bus Selector9/1 -> BusbarTempDiffFltDet/3(LbCDP_AnyBusbarTempVld_flg)  "<LbCDP_AnyBusbarTempVld_flg>"
  Bus Selector9/2 -> BusbarTempDiffFltDet/4(GcCDP_MaxBusbarTemp_C)  "<GcCDP_MaxBusbarTemp_C>"
  Bus Selector9/3 -> BusbarTempDiffFltDet/5(GcCDP_MinBusbarTemp_C)  "<GcCDP_MinBusbarTemp_C>"
  BusbarTempDiffFltDet/1(GbCDP_BusbarTempDiffFltLv2_flg) -> GbCDP_BusbarTempDiffFltLv2_flg/1
  BusbarTempDiffFltDet/2(GbCDP_BusbarTempDiffFltLv1_flg) -> GbCDP_BusbarTempDiffFltLv1_flg/1

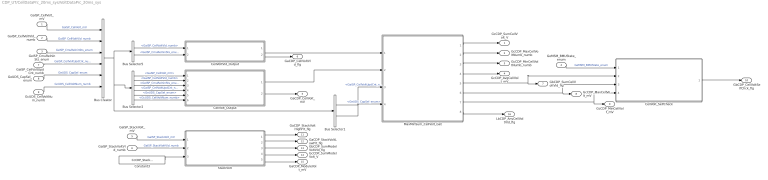
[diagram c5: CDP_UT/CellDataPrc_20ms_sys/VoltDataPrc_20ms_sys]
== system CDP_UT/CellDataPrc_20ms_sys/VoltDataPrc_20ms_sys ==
  GaISP_CellVolt_mV : Inport
  GaISP_CellVoltVld_numb : Inport  Port=2
  GeISP_CmuReIninSts_enum : Inport  Port=3
  GeMSM_BMUState_enum : Inport  Port=4
  GaISP_StackVolt_mV : Inport  Port=5
  GaISP_StackVoltVld_numb : Inport  Port=6
  GaISP_CellVoltUpdCnt_numb : Inport  Port=7
  GeUDS_CapSel_enum : Inport  Port=8
  GcUDS_CellVoltNum_numb : Inport  Port=9
  Bus Creator : BusCreator  Inputs=6
  Bus Selector1 : BusSelector  OutputSignals=GaISP_CellVoltUpdCnt_numb,GeUDS_CapSel_enum
  Bus Selector2 : BusSelector  OutputSignals=GaISP_CellVolt_mV,GaISP_CellVoltVld_numb,GeISP_CmuReIninSts_enum,GaISP_CellVoltUpdCnt_numb,GeUDS_CapSel_enum,GcUDS_CellVoltNum_numb
  Bus Selector5 : BusSelector  OutputSignals=GaISP_CellVoltVld_numb,GeISP_CmuReIninSts_enum
  CellVoltVld_Output : Subsystem
  CellVolt_Output : Subsystem
  CellVolt_SelfCheck : Subsystem
  Constant3 : Constant  Value=CcCDP_StackVoltConfig_numb
  MaxMinSum_CellVolt_Get : Subsystem
  StackVolt : Subsystem
  GcCDP_SumCellVolt_V : Outport
  GcCDP_MaxCellVoltNumb_numb : Outport  Port=2
  GcCDP_MinCellVoltNumb_numb : Outport  Port=3
  GcCDP_AvgCellVolt_mV : Outport  Port=4
  GaCDP_CellVolt_mV : Outport  Port=5
  GaCDP_CellVoltVld_flg : Outport  Port=6
  GbCDP_SumCellVoltVld_flg : Outport  Port=7
  GcCDP_MaxCellVolt_mV : Outport  Port=8
  GcCDP_MinCellVolt_mV : Outport  Port=9
  GbCDP_CellVoltSelfChck_flg : Outport  Port=10
  GaCDP_StackVoltHighFlt_flg : Outport  Port=11
  GaCDP_StackVoltLowFlt_flg : Outport  Port=12
  GbCDP_SumModelVoltVld_flg : Outport  Port=13
  GcCDP_SumModelVolt_V : Outport  Port=14
  GaCDP_ModuleVolt_mV : Outport  Port=15
  LbCDP_AnyCellVoltVld_flg : Outport  Port=16
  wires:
  MaxMinSum_CellVolt_Get/4(GcCDP_AvgCellVolt_mV) -> GcCDP_AvgCellVolt_mV/1
  GaISP_CellVoltVld_numb/1 -> Bus Creator/2  "GaISP_CellVoltVld_numb"
  MaxMinSum_CellVolt_Get/1(GcCDP_SumCellVolt_V) -> GcCDP_SumCellVolt_V/1
  Bus Selector2/1 -> CellVolt_Output/1(GaISP_CellVolt_mV)  "<GaISP_CellVolt_mV>"
  Bus Selector5/1 -> CellVoltVld_Output/1(GaISP_CellVoltVld_numb)  "<GaISP_CellVoltVld_numb>"
  GaISP_CellVolt_mV/1 -> Bus Creator/1  "GaISP_CellVolt_mV"
  MaxMinSum_CellVolt_Get/6(GcCDP_MaxCellVolt_mV) -> GcCDP_MaxCellVolt_mV/1, CellVolt_SelfCheck/3(GcCDP_MaxCellVolt_mV)
  MaxMinSum_CellVolt_Get/5(GbCDP_SumCellVoltVld_flg) -> GbCDP_SumCellVoltVld_flg/1, CellVolt_SelfCheck/2(GbCDP_SumCellVoltVld_flg)
  Bus Selector2/2 -> CellVolt_Output/2(GaISP_CellVoltVld_numb)  "<GaISP_CellVoltVld_numb>"
  Bus Selector5/2 -> CellVoltVld_Output/2(GeISP_CmuReIninSts_enum)  "<GeISP_CmuReIninSts_enum>"
  Bus Creator/1 -> Bus Selector5/1, Bus Selector2/1, Bus Selector1/1
  MaxMinSum_CellVolt_Get/2(GcCDP_MaxCellVoltNumb_numb) -> GcCDP_MaxCellVoltNumb_numb/1
  GeISP_CmuReIninSts_enum/1 -> Bus Creator/3  "GeISP_CmuReIninSts_enum"
  MaxMinSum_CellVolt_Get/3(GcCDP_MinCellVoltNumb_numb) -> GcCDP_MinCellVoltNumb_numb/1
  Bus Selector2/3 -> CellVolt_Output/3(GeISP_CmuReIninSts_enum)  "<GeISP_CmuReIninSts_enum>"
  MaxMinSum_CellVolt_Get/7(GcCDP_MinCellVolt_mV) -> GcCDP_MinCellVolt_mV/1, CellVolt_SelfCheck/4(GcCDP_MinCellVolt_mV)
  CellVolt_SelfCheck/1(GbCDP_CellVoltSelfChck_flg) -> GbCDP_CellVoltSelfChck_flg/1
  CellVoltVld_Output/2(GaCDP_CellVoltVld_flg) -> GaCDP_CellVoltVld_flg/1
  CellVolt_Output/2(GaCDP_CellVolt_mV) -> GaCDP_CellVolt_mV/1
  GeMSM_BMUState_enum/1 -> CellVolt_SelfCheck/1(GeMSM_BMUState_enum)  "GeMSM_BMUState_enum"
  GaISP_StackVolt_mV/1 -> StackVolt/1(GaISP_StackVolt_mV)  "GaISP_StackVolt_mV"
  GaISP_StackVoltVld_numb/1 -> StackVolt/2(GaISP_StackVoltVld_numb)  "GaISP_StackVoltVld_numb"
  StackVolt/1(GaCDP_StackVoltHighFlt_flg) -> GaCDP_StackVoltHighFlt_flg/1
  StackVolt/2(GaCDP_StackVoltLowFlt_flg) -> GaCDP_StackVoltLowFlt_flg/1
  StackVolt/3(GbCDP_SumModelVoltVld_flg) -> GbCDP_SumModelVoltVld_flg/1
  StackVolt/4(GcCDP_SumModelVolt_V) -> GcCDP_SumModelVolt_V/1
  Constant3/1 -> StackVolt/3(CcCDP_StackVoltConfig_numb)
  CellVoltVld_Output/1(LaCDP_CellVoltVld_flg) -> MaxMinSum_CellVolt_Get/1(LaCDP_CellVoltVld_flg)
  CellVolt_Output/1(LaCDP_CellVolt_mV) -> MaxMinSum_CellVolt_Get/2(LaCDP_CellVolt_mV)
  StackVolt/5(GaCDP_ModuleVolt_mV) -> GaCDP_ModuleVolt_mV/1
  MaxMinSum_CellVolt_Get/8(LbCDP_AnyCellVoltVld_flg) -> LbCDP_AnyCellVoltVld_flg/1
  GaISP_CellVoltUpdCnt_numb/1 -> Bus Creator/4  "GaISP_CellVoltUpdCnt_numb"
  GeUDS_CapSel_enum/1 -> Bus Creator/5  "GeUDS_CapSel_enum"
  Bus Selector1/1 -> MaxMinSum_CellVolt_Get/3(GaISP_CellVoltUpdCnt_numb)  "<GaISP_CellVoltUpdCnt_numb>"
  Bus Selector1/2 -> MaxMinSum_CellVolt_Get/4(GeUDS_CapSel_enum)  "<GeUDS_CapSel_enum>"
  Bus Selector2/4 -> CellVolt_Output/4(GaISP_CellVoltUpdCnt_numb)  "<GaISP_CellVoltUpdCnt_numb>"
  Bus Selector2/5 -> CellVolt_Output/5(GeUDS_CapSel_enum)  "<GeUDS_CapSel_enum>"
  GcUDS_CellVoltNum_numb/1 -> Bus Creator/6  "GcUDS_CellVoltNum_numb"
  Bus Selector2/6 -> CellVolt_Output/6(GcUDS_CellVoltNum_numb)  "<GcUDS_CellVoltNum_numb>"

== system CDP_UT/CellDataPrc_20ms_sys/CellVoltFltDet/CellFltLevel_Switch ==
  GcCDP_MinCellTemp_C : Inport
  GeUDS_CapSel_enum : Inport  Port=2
  Bus Creator : BusCreator  Inputs=2
  Bus Selector{,1..5} (6 alike) : BusSelector  OutputSignals=GeUDS_CapSel_enum,LcCDP_MinCellTemp_C
  CDP_2D_Config_Word : AIWAYS_Powertrain_BMS_lib/Signals/2D_Config_Word  Default_Cal_Breakpoint1_Name=CaCDP_CellHighFlt1TempTable_C  Default_Cal_Table1_Name=CaCDP_CATL177CellHighFlt1VoltTable_mV  CATL153Ah_Cal_Breakpoint1_Name=CaCDP_CellHighFlt1TempTable_C  CATL153Ah_Cal_Table1_Name=CaCDP_CATL177CellHighFlt1VoltTable_mV  CATL180Ah_Cal_Breakpoint1_Name=CaCDP_CellHighFlt1TempTable_C  CATL180Ah_Cal_Table1_Name=CaCDP_CATL177CellHighFlt1VoltTable_mV  CATL177Ah_Cal_Breakpoint1_Name=CaCDP_CellHighFlt1TempTable_C  CATL177Ah_Cal_Table1_Name=CaCDP_CATL177CellHighFlt1VoltTable_mV  CATL203Ah_Cal_Breakpoint1_Name=CaCDP_CellHighFlt1TempTable_C  CATL203Ah_Cal_Table1_Name=CaCDP_CATL177CellHighFlt1VoltTable_mV  CATL51Ah_Cal_Breakpoint1_Name=CaCDP_CellHighFlt1TempTable_C  CATL51Ah_Cal_Table1_Name=CaCDP_CATL177CellHighFlt1VoltTable_mV  CATL132Ah_Cal_Breakpoint1_Name=CaCDP_CellHighFlt1TempTable_C  CATL132Ah_Cal_Table1_Name=CaCDP_CATL177CellHighFlt1VoltTable_mV  XWD75Ah_Cal_Breakpoint1_Name=CaCDP_CellHighFlt1TempTable_C  XWD75Ah_Cal_Table1_Name=CaCDP_XWD75CellHighFlt1VoltTable_mV  TFE177Ah_Cal_Breakpoint1_Name=CaCDP_CellHighFlt1TempTable_C  TFE177Ah_Cal_Table1_Name=CaCDP_CATL177CellHighFlt1VoltTable_mV  CATLCTP248Ah_Cal_Breakpoint1_Name=CaCDP_CellHighFlt1TempTable_C  CATLCTP248Ah_Cal_Table1_Name=CaCDP_CATL177CellHighFlt1VoltTable_mV
  CDP_2D_Config_Word1 : AIWAYS_Powertrain_BMS_lib/Signals/2D_Config_Word  Default_Cal_Breakpoint1_Name=CaCDP_CellHighFlt2TempTable_C  Default_Cal_Table1_Name=CaCDP_CATL177CellHighFlt2VoltTable_mV  CATL153Ah_Cal_Breakpoint1_Name=CaCDP_CellHighFlt2TempTable_C  CATL153Ah_Cal_Table1_Name=CaCDP_CATL177CellHighFlt2VoltTable_mV  CATL180Ah_Cal_Breakpoint1_Name=CaCDP_CellHighFlt2TempTable_C  CATL180Ah_Cal_Table1_Name=CaCDP_CATL177CellHighFlt2VoltTable_mV  CATL177Ah_Cal_Breakpoint1_Name=CaCDP_CellHighFlt2TempTable_C  CATL177Ah_Cal_Table1_Name=CaCDP_CATL177CellHighFlt2VoltTable_mV  CATL203Ah_Cal_Breakpoint1_Name=CaCDP_CellHighFlt2TempTable_C  CATL203Ah_Cal_Table1_Name=CaCDP_CATL177CellHighFlt2VoltTable_mV  CATL51Ah_Cal_Breakpoint1_Name=CaCDP_CellHighFlt2TempTable_C  CATL51Ah_Cal_Table1_Name=CaCDP_CATL177CellHighFlt2VoltTable_mV  CATL132Ah_Cal_Breakpoint1_Name=CaCDP_CellHighFlt2TempTable_C  CATL132Ah_Cal_Table1_Name=CaCDP_CATL177CellHighFlt2VoltTable_mV  XWD75Ah_Cal_Breakpoint1_Name=CaCDP_CellHighFlt2TempTable_C  XWD75Ah_Cal_Table1_Name=CaCDP_XWD75CellHighFlt2VoltTable_mV  TFE177Ah_Cal_Breakpoint1_Name=CaCDP_CellHighFlt2TempTable_C  TFE177Ah_Cal_Table1_Name=CaCDP_CATL177CellHighFlt2VoltTable_mV  CATLCTP248Ah_Cal_Breakpoint1_Name=CaCDP_CellHighFlt2TempTable_C  CATLCTP248Ah_Cal_Table1_Name=CaCDP_CATL177CellHighFlt2VoltTable_mV
  CDP_2D_Config_Word2 : AIWAYS_Powertrain_BMS_lib/Signals/2D_Config_Word  Default_Cal_Breakpoint1_Name=CaCDP_CellHighFlt3TempTable_C  Default_Cal_Table1_Name=CaCDP_CATL177CellHighFlt3VoltTable_mV  CATL153Ah_Cal_Breakpoint1_Name=CaCDP_CellHighFlt3TempTable_C  CATL153Ah_Cal_Table1_Name=CaCDP_CATL177CellHighFlt3VoltTable_mV  CATL180Ah_Cal_Breakpoint1_Name=CaCDP_CellHighFlt3TempTable_C  CATL180Ah_Cal_Table1_Name=CaCDP_CATL177CellHighFlt3VoltTable_mV  CATL177Ah_Cal_Breakpoint1_Name=CaCDP_CellHighFlt3TempTable_C  CATL177Ah_Cal_Table1_Name=CaCDP_CATL177CellHighFlt3VoltTable_mV  CATL203Ah_Cal_Breakpoint1_Name=CaCDP_CellHighFlt3TempTable_C  CATL203Ah_Cal_Table1_Name=CaCDP_CATL177CellHighFlt3VoltTable_mV  CATL51Ah_Cal_Breakpoint1_Name=CaCDP_CellHighFlt3TempTable_C  CATL51Ah_Cal_Table1_Name=CaCDP_CATL177CellHighFlt3VoltTable_mV  CATL132Ah_Cal_Breakpoint1_Name=CaCDP_CellHighFlt3TempTable_C  CATL132Ah_Cal_Table1_Name=CaCDP_CATL177CellHighFlt3VoltTable_mV  XWD75Ah_Cal_Breakpoint1_Name=CaCDP_CellHighFlt3TempTable_C  XWD75Ah_Cal_Table1_Name=CaCDP_XWD75CellHighFlt3VoltTable_mV  TFE177Ah_Cal_Breakpoint1_Name=CaCDP_CellHighFlt3TempTable_C  TFE177Ah_Cal_Table1_Name=CaCDP_CATL177CellHighFlt3VoltTable_mV  CATLCTP248Ah_Cal_Breakpoint1_Name=CaCDP_CellHighFlt3TempTable_C  CATLCTP248Ah_Cal_Table1_Name=CaCDP_CATL177CellHighFlt3VoltTable_mV
  CDP_2D_Config_Word3 : AIWAYS_Powertrain_BMS_lib/Signals/2D_Config_Word  Default_Cal_Breakpoint1_Name=CaCDP_CellLowFlt1TempTable_C  Default_Cal_Table1_Name=CaCDP_CATL177CellLowFlt1VoltTable_mV  CATL153Ah_Cal_Breakpoint1_Name=CaCDP_CellLowFlt1TempTable_C  CATL153Ah_Cal_Table1_Name=CaCDP_CATL177CellLowFlt1VoltTable_mV  CATL180Ah_Cal_Breakpoint1_Name=CaCDP_CellLowFlt1TempTable_C  CATL180Ah_Cal_Table1_Name=CaCDP_CATL177CellLowFlt1VoltTable_mV  CATL177Ah_Cal_Breakpoint1_Name=CaCDP_CellLowFlt1TempTable_C  CATL177Ah_Cal_Table1_Name=CaCDP_CATL177CellLowFlt1VoltTable_mV  CATL203Ah_Cal_Breakpoint1_Name=CaCDP_CellLowFlt1TempTable_C  CATL203Ah_Cal_Table1_Name=CaCDP_CATL177CellLowFlt1VoltTable_mV  CATL51Ah_Cal_Breakpoint1_Name=CaCDP_CellLowFlt1TempTable_C  CATL51Ah_Cal_Table1_Name=CaCDP_CATL177CellLowFlt1VoltTable_mV  CATL132Ah_Cal_Breakpoint1_Name=CaCDP_CellLowFlt1TempTable_C  CATL132Ah_Cal_Table1_Name=CaCDP_CATL177CellLowFlt1VoltTable_mV  XWD75Ah_Cal_Breakpoint1_Name=CaCDP_CellLowFlt1TempTable_C  XWD75Ah_Cal_Table1_Name=CaCDP_XWD75CellLowFlt1VoltTable_mV  TFE177Ah_Cal_Breakpoint1_Name=CaCDP_CellLowFlt1TempTable_C  TFE177Ah_Cal_Table1_Name=CaCDP_CATL177CellLowFlt1VoltTable_mV  CATLCTP248Ah_Cal_Breakpoint1_Name=CaCDP_CellLowFlt1TempTable_C  CATLCTP248Ah_Cal_Table1_Name=CaCDP_CATL177CellLowFlt1VoltTable_mV
  CDP_2D_Config_Word4 : AIWAYS_Powertrain_BMS_lib/Signals/2D_Config_Word  Default_Cal_Breakpoint1_Name=CaCDP_CellLowFlt2TempTable_C  Default_Cal_Table1_Name=CaCDP_CATL177CellLowFlt2VoltTable_mV  CATL153Ah_Cal_Breakpoint1_Name=CaCDP_CellLowFlt2TempTable_C  CATL153Ah_Cal_Table1_Name=CaCDP_CATL177CellLowFlt2VoltTable_mV  CATL180Ah_Cal_Breakpoint1_Name=CaCDP_CellLowFlt2TempTable_C  CATL180Ah_Cal_Table1_Name=CaCDP_CATL177CellLowFlt2VoltTable_mV  CATL177Ah_Cal_Breakpoint1_Name=CaCDP_CellLowFlt2TempTable_C  CATL177Ah_Cal_Table1_Name=CaCDP_CATL177CellLowFlt2VoltTable_mV  CATL203Ah_Cal_Breakpoint1_Name=CaCDP_CellLowFlt2TempTable_C  CATL203Ah_Cal_Table1_Name=CaCDP_CATL177CellLowFlt2VoltTable_mV  CATL51Ah_Cal_Breakpoint1_Name=CaCDP_CellLowFlt2TempTable_C  CATL51Ah_Cal_Table1_Name=CaCDP_CATL177CellLowFlt2VoltTable_mV  CATL132Ah_Cal_Breakpoint1_Name=CaCDP_CellLowFlt2TempTable_C  CATL132Ah_Cal_Table1_Name=CaCDP_CATL177CellLowFlt2VoltTable_mV  XWD75Ah_Cal_Breakpoint1_Name=CaCDP_CellLowFlt2TempTable_C  XWD75Ah_Cal_Table1_Name=CaCDP_XWD75CellLowFlt2VoltTable_mV  TFE177Ah_Cal_Breakpoint1_Name=CaCDP_CellLowFlt2TempTable_C  TFE177Ah_Cal_Table1_Name=CaCDP_CATL177CellLowFlt2VoltTable_mV  CATLCTP248Ah_Cal_Breakpoint1_Name=CaCDP_CellLowFlt2TempTable_C  CATLCTP248Ah_Cal_Table1_Name=CaCDP_CATL177CellLowFlt2VoltTable_mV
  CDP_2D_Config_Word5 : AIWAYS_Powertrain_BMS_lib/Signals/2D_Config_Word  Default_Cal_Breakpoint1_Name=CaCDP_CellLowFlt3TempTable_C  Default_Cal_Table1_Name=CaCDP_CATL177CellLowFlt3VoltTable_mV  CATL153Ah_Cal_Breakpoint1_Name=CaCDP_CellLowFlt3TempTable_C  CATL153Ah_Cal_Table1_Name=CaCDP_CATL177CellLowFlt3VoltTable_mV  CATL180Ah_Cal_Breakpoint1_Name=CaCDP_CellLowFlt3TempTable_C  CATL180Ah_Cal_Table1_Name=CaCDP_CATL177CellLowFlt3VoltTable_mV  CATL177Ah_Cal_Breakpoint1_Name=CaCDP_CellLowFlt3TempTable_C  CATL177Ah_Cal_Table1_Name=CaCDP_CATL177CellLowFlt3VoltTable_mV  CATL203Ah_Cal_Breakpoint1_Name=CaCDP_CellLowFlt3TempTable_C  CATL203Ah_Cal_Table1_Name=CaCDP_CATL177CellLowFlt3VoltTable_mV  CATL51Ah_Cal_Breakpoint1_Name=CaCDP_CellLowFlt3TempTable_C  CATL51Ah_Cal_Table1_Name=CaCDP_CATL177CellLowFlt3VoltTable_mV  CATL132Ah_Cal_Breakpoint1_Name=CaCDP_CellLowFlt3TempTable_C  CATL132Ah_Cal_Table1_Name=CaCDP_CATL177CellLowFlt3VoltTable_mV  XWD75Ah_Cal_Breakpoint1_Name=CaCDP_CellLowFlt3TempTable_C  XWD75Ah_Cal_Table1_Name=CaCDP_XWD75CellLowFlt3VoltTable_mV  TFE177Ah_Cal_Breakpoint1_Name=CaCDP_CellLowFlt3TempTable_C  TFE177Ah_Cal_Table1_Name=CaCDP_CATL177CellLowFlt3VoltTable_mV  CATLCTP248Ah_Cal_Breakpoint1_Name=CaCDP_CellLowFlt3TempTable_C  CATLCTP248Ah_Cal_Table1_Name=CaCDP_CATL177CellLowFlt3VoltTable_mV
  Data Type Conversion : DataTypeConversion  OutDataTypeStr=fixdt(0,8,1,-40)
  LcCDP_CellHighFltLevel1_mV : Outport
  LcCDP_CellHighFltLevel2_mV : Outport  Port=2
  LcCDP_CellHighFltLevel3_mV : Outport  Port=3
  LcCDP_CellLowFltLevel1_mV : Outport  Port=4
  LcCDP_CellLowFltLevel2_mV : Outport  Port=5
  LcCDP_CellLowFltLevel3_mV : Outport  Port=6
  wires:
  CDP_2D_Config_Word/1 -> LcCDP_CellHighFltLevel1_mV/1  "LcCDP_CellHighFltLevel1_mV"
  GcCDP_MinCellTemp_C/1 -> Data Type Conversion/1
  CDP_2D_Config_Word1/1 -> LcCDP_CellHighFltLevel2_mV/1  "LcCDP_CellHighFltLevel2_mV"
  CDP_2D_Config_Word2/1 -> LcCDP_CellHighFltLevel3_mV/1  "LcCDP_CellHighFltLevel3_mV"
  CDP_2D_Config_Word3/1 -> LcCDP_CellLowFltLevel1_mV/1  "LcCDP_CellLowFltLevel1_mV"
  CDP_2D_Config_Word4/1 -> LcCDP_CellLowFltLevel2_mV/1  "LcCDP_CellLowFltLevel2_mV"
  CDP_2D_Config_Word5/1 -> LcCDP_CellLowFltLevel3_mV/1  "LcCDP_CellLowFltLevel3_mV"
  Data Type Conversion/1 -> Bus Creator/1  "LcCDP_MinCellTemp_C"
  GeUDS_CapSel_enum/1 -> Bus Creator/2
  Bus Creator/1 -> Bus Selector2/1, Bus Selector3/1, Bus Selector5/1, Bus Selector4/1, Bus Selector1/1, Bus Selector/1
  Bus Selector/1 -> CDP_2D_Config_Word/1  "<GeUDS_CapSel_enum>"
  Bus Selector/2 -> CDP_2D_Config_Word/2  "<LcCDP_MinCellTemp_C>"
  Bus Selector1/1 -> CDP_2D_Config_Word1/1  "<GeUDS_CapSel_enum>"
  Bus Selector1/2 -> CDP_2D_Config_Word1/2  "<LcCDP_MinCellTemp_C>"
  Bus Selector2/1 -> CDP_2D_Config_Word2/1  "<GeUDS_CapSel_enum>"
  Bus Selector2/2 -> CDP_2D_Config_Word2/2  "<LcCDP_MinCellTemp_C>"
  Bus Selector3/1 -> CDP_2D_Config_Word3/1  "<GeUDS_CapSel_enum>"
  Bus Selector3/2 -> CDP_2D_Config_Word3/2  "<LcCDP_MinCellTemp_C>"
  Bus Selector4/1 -> CDP_2D_Config_Word4/1  "<GeUDS_CapSel_enum>"
  Bus Selector4/2 -> CDP_2D_Config_Word4/2  "<LcCDP_MinCellTemp_C>"
  Bus Selector5/1 -> CDP_2D_Config_Word5/1  "<GeUDS_CapSel_enum>"
  Bus Selector5/2 -> CDP_2D_Config_Word5/2  "<LcCDP_MinCellTemp_C>"
